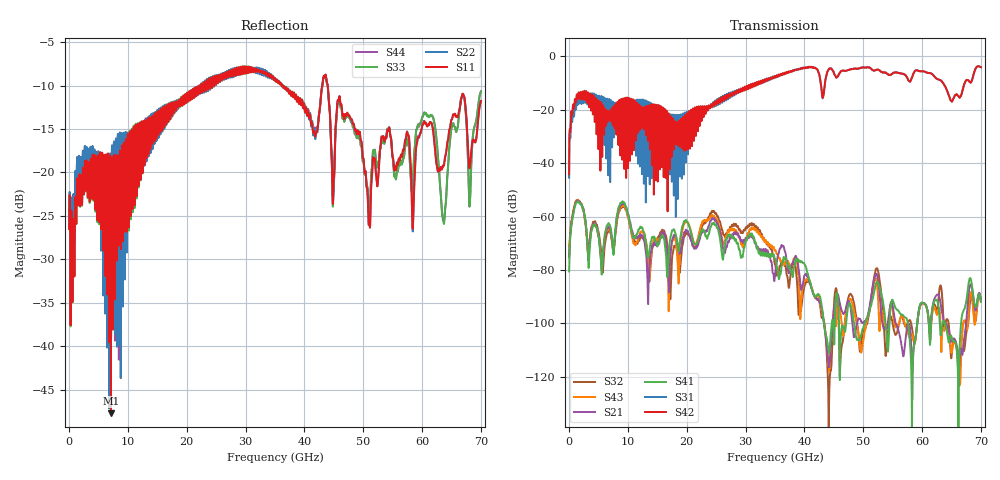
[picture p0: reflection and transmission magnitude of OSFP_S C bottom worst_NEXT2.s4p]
! AWR Design Environment (8415) Mon Jan 07 17:45:50 2019
! Document = 'OSFP Channel_S'
! nPorts: 4, nXvals: 7001
# HZ S DB R 50
!Freq DBS11 AngS11 DBS12 AngS12 DBS13 AngS13 DBS14 AngS14
!	DBS21 AngS21 DBS22 AngS22 DBS23 AngS23 DBS24 AngS24
!	DBS31 AngS31 DBS32 AngS32 DBS33 AngS33 DBS34 AngS34
!	DBS41 AngS41 DBS42 AngS42 DBS43 AngS43 DBS44 AngS44
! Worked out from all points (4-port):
!   7000 points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, 10 MHz to 70 GHz, reference 50 ohm
!   strongest paths, dB at 10 MHz, 17.51 GHz, 35.01 GHz, 52.51 GHz, 70 GHz:
!     S42: -44.1, -26.6, -7.4, -4.9, -4.0
!     S31: -45.4, -29.5, -7.4, -4.9, -4.0
!     S41: -80.5, -65.2, -76.0, -84.7, -91.9
!     S21: -75.2, -68.8, -81.8, -83.7, -91.3
!     S43: -70.9, -69.4, -72.7, -89.9, -91.8
!     S32: -74.3, -75.3, -78.0, -80.3, -91.2
!   lowest |S11| = -47.7 dB at 7.12 GHz (marker M1), VSWR 1.01, Z = 50.1 - j0.408 ohm
!   |S11| at or under -10 dB: start of sweep to 22.43 GHz; 36.33 GHz to 43.05 GHz (6.718 GHz wide, 16.9 % of centre); 43.97 GHz to end of sweep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
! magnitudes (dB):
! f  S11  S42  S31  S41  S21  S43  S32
! 10 MHz  -26.5  -44.1  -45.4  -80.5  -75.2  -70.9  -74.3
! 1.43 GHz  -20.8  -15.6  -17.3  -54.4  -54.0  -53.8  -53.7
! 3.33 GHz  -18.9  -15.8  -14.9  -79.2  -75.8  -73.3  -74.7
! 7.12 GHz  -47.7  -24.2  -16.7  -64.8  -65.8  -66.5  -66.6
! 30.86 GHz  -7.9  -10.5  -10.7  -67.0  -67.5  -65.1  -63.2
! 63.64 GHz  -19.2  -10.2  -10.1  -99.1  -98.6  -102.4  -99.0
! 70 GHz  -11.8  -4.0  -4.0  -91.9  -91.3  -91.8  -91.2
